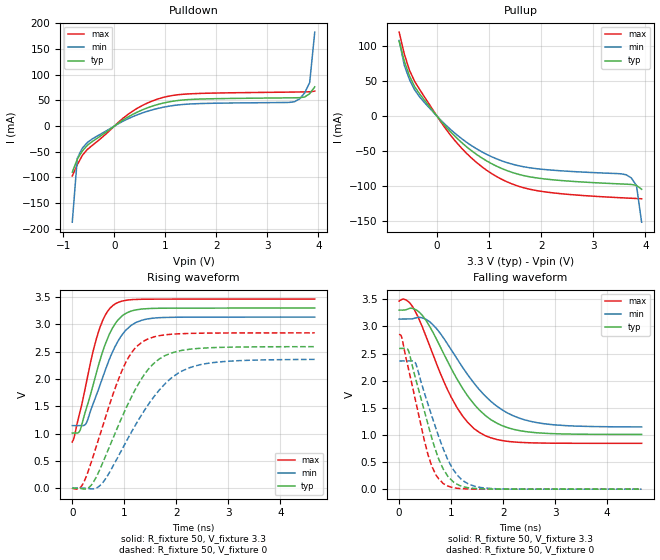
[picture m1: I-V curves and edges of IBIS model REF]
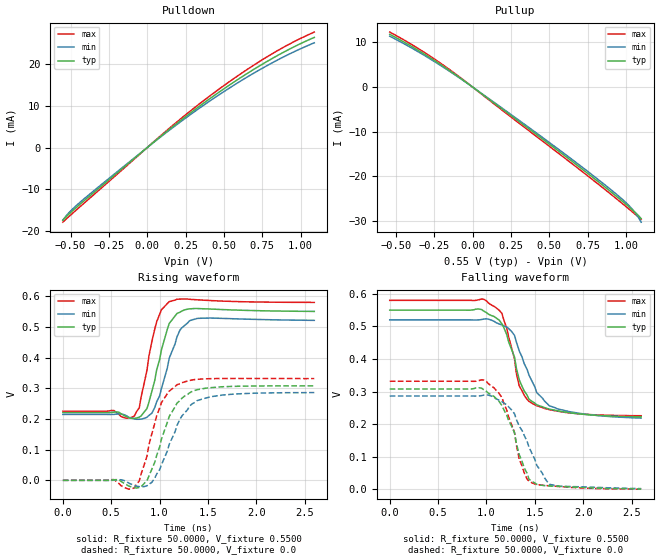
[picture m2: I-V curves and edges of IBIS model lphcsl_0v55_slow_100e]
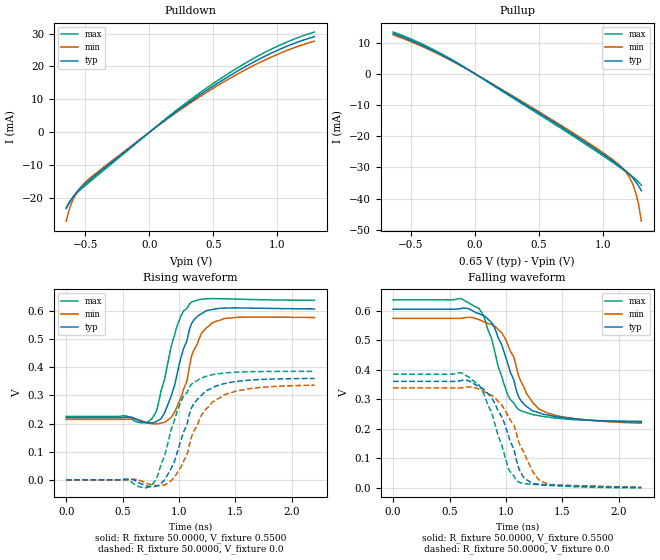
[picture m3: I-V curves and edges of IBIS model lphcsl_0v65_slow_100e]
| Integrated Devices Technolgy, Inc
[IBIS Ver]   4.1
[File name]   9fgl06p1.ibs
[File Rev]   1.0
|Rev history   1.0   original ibis data
[Date]   22 March, 2016
[Disclaimer] Integrated Device Technology, Inc. ("IDT") hereby grants the
   user of this ibis model a non-exclusive, nontransferable
   license to use this ibis model under the following terms. the
   user is granted this license only to use the ibis model and is
   not granted rights to sell, copy (except as needed to run the
   ibis model), rent, lease or sub-license the ibis model in
   whole or in part, or in modified form to anyone. the user may
   modify the ibis model to suit its specific applications, but
   rights to derivative works and such modifications shall belong
   to idt. this ibis model is provided on an as is" basis and idt
   makes absolutely no warranty with respect to the information
   contained herein. idt disclaims and customer waives all
   warranties, express and implied, including warranties of
   merchantability and fitness for a particular purpose. the
   entire risk as to quality and performance is with the user
   accordingly, in no event shall idt be liable for any direct or
   indirect damages, whether in contract or tort, including any
   lost profits or other incidental, consequential, exemplary, or
   punitive damages arising out of the use or application of the
   ibis model. further, idt reserves the right to make changes
   without notice to any product herein to improve reliability,
   function, or design. idt does not convey any license under
   patent rights or any other intellectual property rights,
   including those of third parties. idt is not obligated to
   provide maintenance or support for the licensed ibis model.
[Copyright]   Copyright 2012, Integrated Devices Technolgy, Inc. all rights
   reserved
[Component]   9fgl06p1
[Manufacturer] Integrated Device Technology, Inc.
[Package]
R_pkg   72.4655m   58.886m   86.045m
L_pkg   1.47175nH   1.11650nH   1.77850nH
C_pkg   0.07747pF   0.07444pF   0.08050pF
[Pin] signal_name  model_name
1   vSS_EN_tri   GND
2   X1_25   X1
3   X2   X2
4   VDDXTAL3.3   POWER
5   VDDREF3.3   POWER
6   vSADR/REF3.3   REF
7   NC   NC
8   GNDDIG   GND
9   SCLK_3.3   SCIN
10   SDATA_3.3   SCIN
11   VDDDIG3.3   POWER
12   VDDIO   POWER
13   vOE0#   IN
14   DIF0   LP_HCSL
15   DIF0#   LP_HCSL
16   VDD3.3   POWER
17   VDDIO   POWER
18   DIF1   LP_HCSL
19   DIF1#   LP_HCSL
20   NC   NC
21   vOE1#   IN
22   DIF2   LP_HCSL
23   DIF2#   LP_HCSL
24   vOE2#   IN
25   NC   NC
26   VDDA3.3   POWER
27   VDDIO   POWER
28   DIF3   LP_HCSL
29   DIF3#   LP_HCSL
30   vOE3#   IN
31   VDD3.3   POWER
32   VDDIO   POWER
33   DIF4   LP_HCSL
34   DIF4#   LP_HCSL
35   vOE4#   IN
36   DIF5   LP_HCSL
37   DIF5#   LP_HCSL
38   vOE5#   IN
39   VDDIO   POWER
40   ^CKPWRGD_PD#   PD
41   ePAD   GND
[Diff Pin]  inv_pin  vdiff tdelay_typ tdelay_min  tdelay_max
14   15   NA   0   0   0
18   19   NA   0   0   0
22   23   NA   0   0   0
28   29   NA   0   0   0
33   34   NA   0   0   0
36   37   NA   0   0   0
[Model Selector] LP_HCSL
lphcsl_0v55_fast_33e amplitude 0.55V, slew rate fast, 33 ohm diff impedance
lphcsl_0v55_slow_33e amplitude 0.55V, slew rate slow, 33 ohm diff impedance
lphcsl_0v65_fast_33e amplitude 0.65V, slew rate fast, 33 ohm diff impedance
lphcsl_0v65_slow_33e amplitude 0.65V, slew rate slow, 33 ohm diff impedance
lphcsl_0v70_fast_33e amplitude 0.70V, slew rate fast, 33 ohm diff impedance
lphcsl_0v70_slow_33e amplitude 0.70V, slew rate slow, 33 ohm diff impedance
lphcsl_0v80_fast_33e amplitude 0.80V, slew rate fast, 33 ohm diff impedance
lphcsl_0v80_slow_33e amplitude 0.80V, slew rate slow, 33 ohm diff impedance
lphcsl_0v55_fast_85e amplitude 0.55V, slew rate fast, 85 ohm diff impedance
lphcsl_0v55_slow_85e amplitude 0.55V, slew rate slow, 85 ohm diff impedance
lphcsl_0v65_fast_85e amplitude 0.65V, slew rate fast, 85 ohm diff impedance
lphcsl_0v65_slow_85e amplitude 0.65V, slew rate slow, 85 ohm diff impedance
lphcsl_0v70_fast_85e amplitude 0.70V, slew rate fast, 85 ohm diff impedance
lphcsl_0v70_slow_85e amplitude 0.70V, slew rate slow, 85 ohm diff impedance
lphcsl_0v80_fast_85e amplitude 0.80V, slew rate fast, 85 ohm diff impedance
lphcsl_0v80_slow_85e amplitude 0.80V, slew rate slow, 85 ohm diff impedance
lphcsl_0v55_fast_100e amplitude 0.55V, slew rate fast, 100 ohm diff impedance
lphcsl_0v55_slow_100e amplitude 0.55V, slew rate slow, 100 ohm diff impedance
lphcsl_0v65_fast_100e amplitude 0.65V, slew rate fast, 100 ohm diff impedance
lphcsl_0v65_slow_100e amplitude 0.65V, slew rate slow, 100 ohm diff impedance
lphcsl_0v70_fast_100e amplitude 0.70V, slew rate fast, 100 ohm diff impedance
lphcsl_0v70_slow_100e amplitude 0.70V, slew rate slow, 100 ohm diff impedance
lphcsl_0v80_fast_100e amplitude 0.80V, slew rate fast, 100 ohm diff impedance
lphcsl_0v80_slow_100e amplitude 0.80V, slew rate slow, 100 ohm diff impedance
| Models and submodels in the file (30): REF (Output), lphcsl_0v55_fast_100e (Output), lphcsl_0v55_slow_100e (Output), lphcsl_0v65_fast_100e (Output), lphcsl_0v65_slow_100e (Output), lphcsl_0v70_fast_100e (Output), lphcsl_0v70_slow_100e (Output), lphcsl_0v80_fast_100e (Output), lphcsl_0v80_slow_100e (Output), lphcsl_0v55_fast_85e (Output), lphcsl_0v55_slow_85e (Output), lphcsl_0v65_fast_85e (Output), lphcsl_0v65_slow_85e (Output), lphcsl_0v70_fast_85e (Output), lphcsl_0v70_slow_85e (Output), lphcsl_0v80_fast_85e (Output), lphcsl_0v80_slow_85e (Output), lphcsl_0v55_fast_33e (Output), lphcsl_0v55_slow_33e (Output), lphcsl_0v65_fast_33e (Output), lphcsl_0v65_slow_33e (Output), lphcsl_0v70_fast_33e (Output), lphcsl_0v70_slow_33e (Output), lphcsl_0v80_fast_33e (Output), lphcsl_0v80_slow_33e (Output), SCIN (Input), IN (Input), PD (Input), X1 (Input), X2 (Output)
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[Model]   REF
Model_type   Output
Polarity   Non-Inverting
|   typ   min   max
C_comp   2pF   1.5pF   2.5pF
Vmeas = 1.65V
Rref = 50
Cref = 0
Vref = 1.65V
|   typ   min   max
[Voltage range]   3.3V   3.135V   3.465V
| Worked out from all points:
|   slope of the pulldown table from 0 to 0.495 V, typ, clamps not added: 16.9 ohm
|   slope of the pullup table from 0 to 0.495 V, typ, clamps not added: 12.6 ohm
|   rising waveform, R_fixture 50, V_fixture 3.3: 20-80 % time 450ps typ, 507ps min, 388ps max; typ from 1.01 V to 3.3 V
|   falling waveform, R_fixture 50, V_fixture 3.3: 20-80 % time 857ps typ, 970ps min, 739ps max; typ from 3.3 V to 1.01 V
|   rising waveform, R_fixture 50, V_fixture 0: 20-80 % time 771ps typ, 936ps min, 618ps max; typ from 0 V to 2.59 V
|   falling waveform, R_fixture 50, V_fixture 0: 20-80 % time 472ps typ, 527ps min, 413ps max; typ from 2.59 V to 0 V
[Pulldown]
|Voltage   I (typ)   I (min)   I (max)
|Note, modeling breaks down at 250mA and above.  This is well beyond the functional   |
|operating range of the device.  Should this scenario occur, catastrophic failure and   |
|possible damage to the device and/or board is of higher concern than the I-V curve   |
|behavior.  The IBIS checker will flag currents in excess of 10A with warnings.  Lines   |
|with currents in excess of 0.35 A have been commented out.  The points still remain|
|available to the user if the user desires to use them.   |
|-3.30000e+00   -4.58626e+02   -3.98855e+02   -5.58913e+02
|-3.20100e+00   -4.38670e+02   -3.81813e+02   -5.34126e+02
|-3.10200e+00   -4.18718e+02   -3.64776e+02   -5.09343e+02
|-3.00300e+00   -3.98770e+02   -3.47745e+02   -4.84563e+02
|-2.90400e+00   -3.78827e+02   -3.30720e+02   -4.59787e+02
|-2.80500e+00   -3.58890e+02   -3.13701e+02   -4.35015e+02
|-2.70600e+00   -3.38959e+02   -2.96690e+02   -4.10248e+02
|-2.60700e+00   -3.19035e+02   -2.79688e+02   -3.85486e+02
|-2.50800e+00   -2.99119e+02   -2.62696e+02   -3.60731e+02
|-2.40900e+00   -2.79213e+02   -2.45715e+02   -3.35984e+02
|-2.31000e+00   -2.59319e+02   -2.28747e+02   -3.11245e+02
|-2.21100e+00   -2.39437e+02   -2.11796e+02   -2.86516e+02
|-2.11200e+00   -2.19572e+02   -1.94864e+02   -2.61800e+02
|-2.01300e+00   -1.99726e+02   -1.77955e+02   -2.37100e+02
|-1.91400e+00   -1.79905e+02   -1.61075e+02   -2.12419e+02
|-1.81500e+00   -1.60116e+02   -1.44233e+02   -1.87763e+02
|-1.71600e+00   -1.40369e+02   -1.27441e+02   -1.63140e+02
|-1.61700e+00   -1.20682e+02   -1.10717e+02   -1.38565e+02
|-1.51800e+00   -1.01080e+02   -9.40899e+01   -1.14061e+02
|-1.41900e+00   -8.16135e+01   -7.76121e+01   -8.96701e+01
|-1.32000e+00   -6.23864e+01   -6.13830e+01   -6.54941e+01
|-1.22100e+00   -4.36066e+01   -4.55730e+01   -4.17841e+01
|-1.12200e+00   -2.55446e+01   -3.03740e+01   -1.89497e+01
|-1.02300e+00   -8.13369e+00   -1.57511e+01   -1.01906e+00
|-9.24000e-01   -3.55892e-01   -2.38948e+00   -1.27879e-01
-825mV    -89.74mA   -186.9mA   -97.05mA
-726mV    -64.34mA   -62.46mA   -75.03mA
-627mV    -48.3mA    -42.65mA   -56.86mA
-528mV    -37.22mA   -31.89mA   -45.33mA
363mV     22.88mA    18.45mA    29.33mA
957mV     44.74mA    36.62mA    55.73mA
1.551V    52.05mA    43.3mA     63.04mA
3.531V    55.03mA    47.39mA    66.19mA
3.63V     55.21mA    52.95mA    66.32mA
3.729V    56.59mA    64.36mA    66.46mA
3.828V    63.02mA    84.81mA    66.64mA
3.927V    76.26mA    182.8mA    67.99mA
| 4.02600e+00   9.63336e-02   1.95544e+00   7.56685e-02
| 4.12500e+00   1.29319e-01   1.96109e+01   9.19025e-02
| 4.22400e+00   6.62462e-01   4.21550e+01   1.15435e-01
| 4.32300e+00   1.51637e+01   6.47670e+01   1.37492e-01
| 4.42200e+00   4.22442e+01   8.74545e+01   2.35006e-01
| 4.52100e+00   6.94172e+01   1.10195e+02   8.92943e+00
| 4.62000e+00   9.66780e+01   1.32968e+02   4.35589e+01
| 4.71900e+00   1.23991e+02   1.55761e+02   7.83218e+01
| 4.81800e+00   1.51333e+02   1.78569e+02   1.13180e+02
| 4.91700e+00   1.78693e+02   2.01386e+02   1.48085e+02
| 5.01600e+00   2.06065e+02   2.24210e+02   1.83014e+02
| 5.11500e+00   2.33446e+02   2.47041e+02   2.17958e+02
| 5.21400e+00   2.60834e+02   2.69877e+02   2.52912e+02
| 5.31300e+00   2.88228e+02   2.92717e+02   2.87874e+02
| 5.41200e+00   3.15625e+02   3.15560e+02   3.22841e+02
| 5.51100e+00   3.43027e+02   3.38407e+02   3.57813e+02
| 5.61000e+00   3.70432e+02   3.61256e+02   3.92789e+02
| 5.70900e+00   3.97841e+02   3.84108e+02   4.27769e+02
| 5.80800e+00   4.25252e+02   4.06963e+02   4.62752e+02
| 5.90700e+00   4.52666e+02   4.29821e+02   4.97738e+02
| 6.00600e+00   4.80082e+02   4.52680e+02   5.32727e+02
| 6.10500e+00   5.07501e+02   4.75543e+02   5.67718e+02
| 6.20400e+00   5.34922e+02   4.98407e+02   6.02711e+02
| 6.30300e+00   5.62345e+02   5.21273e+02   6.37705e+02
| 6.40200e+00   5.89770e+02   5.44142e+02   6.72701e+02
| 6.50100e+00   6.17197e+02   5.67013e+02   7.07699e+02
| 6.60000e+00   6.44626e+02   5.89886e+02   7.42698e+02
[Pullup]
|Voltage   I (typ)   I (min)   I (max)
|Note, modeling breaks down at 250mA and above.  This is well beyond the functional   |
|operating range of the device.  Should this scenario occur, catastrophic failure and   |
|possible damage to the device and/or board is of higher concern than the I-V curve   |
|behavior.  The IBIS checker will flag currents in excess of 10A with warnings.  Lines   |
|with currents in excess of 0.35 A have been commented out.  The points still remain|
|available to the user if the user desires to use them.   |
|-3.30000e+00   6.44680e+02   5.51825e+02   8.01095e+02
|-3.20100e+00   6.17254e+02   5.28958e+02   7.66095e+02
|-3.10200e+00   5.89830e+02   5.06093e+02   7.31096e+02
|-3.00300e+00   5.62407e+02   4.83230e+02   6.96098e+02
|-2.90400e+00   5.34987e+02   4.60368e+02   6.61102e+02
|-2.80500e+00   5.07568e+02   4.37509e+02   6.26108e+02
|-2.70600e+00   4.80150e+02   4.14651e+02   5.91115e+02
|-2.60700e+00   4.52735e+02   3.91796e+02   5.56124e+02
|-2.50800e+00   4.25322e+02   3.68942e+02   5.21136e+02
|-2.40900e+00   3.97911e+02   3.46091e+02   4.86149e+02
|-2.31000e+00   3.70503e+02   3.23243e+02   4.51165e+02
|-2.21100e+00   3.43097e+02   3.00397e+02   4.16183e+02
|-2.11200e+00   3.15694e+02   2.77554e+02   3.81204e+02
|-2.01300e+00   2.88295e+02   2.54715e+02   3.46229e+02
|-1.91400e+00   2.60900e+02   2.31881e+02   3.11257e+02
|-1.81500e+00   2.33510e+02   2.09052e+02   2.76290e+02
|-1.71600e+00   2.06127e+02   1.86229e+02   2.41329e+02
|-1.61700e+00   1.78751e+02   1.63415e+02   2.06375e+02
|-1.51800e+00   1.51388e+02   1.40613e+02   1.71432e+02
|-1.41900e+00   1.24042e+02   1.17829e+02   1.36506e+02
|-1.32000e+00   9.67252e+01   9.50724e+01   1.01609e+02
|-1.22100e+00   6.94599e+01   7.23604e+01   6.67700e+01
|-1.12200e+00   4.22820e+01   4.97173e+01   3.20469e+01
|-1.02300e+00   1.51962e+01   2.71494e+01   2.11287e+00
|-9.24000e-01   6.89030e-01   5.34223e+00   1.97623e-01
|-8.25000e-01   1.48916e-01   3.54714e-01   1.54087e-01
-726mV    106.9mA    108.2mA    120.1mA
-627mV    78.63mA    72.64mA    88.74mA
-528mV    57.36mA    52.3mA     65.5mA
-330mV    31.45mA    27.24mA    37.82mA
363mV     -30.02mA   -25.58mA   -36.52mA
957mV     -64.05mA   -54.65mA   -77.43mA
1.353V    -77.99mA   -66.51mA   -94.06mA
1.848V    -87.45mA   -74.38mA   -105.4mA
3.63V     -97.08mA   -83.63mA   -116.9mA
3.729V    -97.47mA   -88.18mA   -117.2mA
3.828V    -98.9mA    -99mA      -117.5mA
3.927V    -104.4mA   -151.4mA   -117.9mA
| 4.02600e+00   -1.15410e-01   -9.65481e-01   -1.19366e-01
| 4.12500e+00   -1.36603e-01   -1.09884e+01   -1.26324e-01
| 4.22400e+00   -3.99361e-01   -2.54841e+01   -1.40663e-01
| 4.32300e+00   -8.17474e+00   -4.04654e+01   -1.58277e-01
| 4.42200e+00   -2.55843e+01   -5.60873e+01   -2.17491e-01
| 4.52100e+00   -4.36450e+01   -7.21990e+01   -4.28595e+00
| 4.62000e+00   -6.24226e+01   -8.86071e+01   -2.64922e+01
| 4.71900e+00   -8.16508e+01   -1.05189e+02   -4.96573e+01
| 4.81800e+00   -1.01115e+02   -1.21884e+02   -7.35635e+01
| 4.91700e+00   -1.20715e+02   -1.38656e+02   -9.78285e+01
| 5.01600e+00   -1.40403e+02   -1.55482e+02   -1.22263e+02
| 5.11500e+00   -1.60149e+02   -1.72350e+02   -1.46794e+02
| 5.21400e+00   -1.79938e+02   -1.89250e+02   -1.71387e+02
| 5.31300e+00   -1.99760e+02   -2.06175e+02   -1.96022e+02
| 5.41200e+00   -2.19606e+02   -2.23121e+02   -2.20688e+02
| 5.51100e+00   -2.39472e+02   -2.40084e+02   -2.45378e+02
| 5.61000e+00   -2.59355e+02   -2.57061e+02   -2.70086e+02
| 5.70900e+00   -2.79251e+02   -2.74051e+02   -2.94808e+02
| 5.80800e+00   -2.99159e+02   -2.91052e+02   -3.19543e+02
| 5.90700e+00   -3.19077e+02   -3.08062e+02   -3.44288e+02
| 6.00600e+00   -3.39003e+02   -3.25080e+02   -3.69042e+02
| 6.10500e+00   -3.58937e+02   -3.42106e+02   -3.93803e+02
| 6.20400e+00   -3.78878e+02   -3.59138e+02   -4.18571e+02
| 6.30300e+00   -3.98826e+02   -3.76177e+02   -4.43346e+02
| 6.40200e+00   -4.18779e+02   -3.93221e+02   -4.68125e+02
| 6.50100e+00   -4.38737e+02   -4.10271e+02   -4.92910e+02
| 6.60000e+00   -4.58699e+02   -4.27325e+02   -5.17700e+02
[Ramp]
|   typ   min   max
dV/dt_r   1.566/0.774n   1.425/0.94n   1.718/0.621n
dV/dt_f   1.396/0.866n   1.212/0.979n   1.595/0.746n
R_load =   50
[Rising Waveform]
R_fixture = 50
V_fixture = 3.3   |Vcc_typ
V_fixture_min = 3.135 |Vcc_min
V_fixture_max = 3.465 |Vcc_max
C_fixture = 0.0p
| Time   typ   min   max
0s        1.008V     1.145V     844.6mV
34.71ps   1.008V     1.145V     923.1mV
154.3ps   1.071V     1.145V     1.413V
275.2ps   1.472V     1.202V     1.956V
479.5ps   2.168V     1.745V     2.789V
635.5ps   2.641V     2.166V     3.174V
823.7ps   3.01V      2.596V     3.375V
1.129ns   3.244V     2.981V     3.453V
1.433ns   3.289V     3.099V     3.463V
4.662ns   3.3V       3.135V     3.465V
[Falling Waveform]
R_fixture = 50
V_fixture = 3.3   |Vcc_typ
V_fixture_min = 3.135 |Vcc_min
V_fixture_max = 3.465 |Vcc_max
C_fixture = 0.0p
| Time   typ   min   max
0s        3.3V       3.135V     3.465V
120.3ps   3.304V     3.135V     3.493V
247.8ps   3.333V     3.138V     3.377V
425ps     3.225V     3.162V     3.038V
624.4ps   2.937V     3.054V     2.545V
1.111ns   2.034V     2.407V     1.506V
1.539ns   1.462V     1.838V     1.048V
1.979ns   1.171V     1.463V     896.3mV
2.515ns   1.052V     1.252V     854.4mV
4.666ns   1.008V     1.146V     844.6mV
[Rising Waveform]
R_fixture = 50
V_fixture = 0
C_fixture = 0.0p
| Time   typ   min   max
0s        23.89nV    60.43nV    30.4nV
191.1ps   -13.44mV   129.7uV    54.48mV
415.8ps   124mV      -13.01mV   625.4mV
623.1ps   548.9mV    147.1mV    1.254V
939.4ps   1.267V     680mV      2.117V
1.156ns   1.708V     1.059V     2.505V
1.348ns   2.027V     1.367V     2.681V
1.787ns   2.43V      1.916V     2.809V
2.339ns   2.554V     2.232V     2.838V
4.662ns   2.593V     2.359V     2.845V
[Falling Waveform]
R_fixture = 50
V_fixture = 0
C_fixture = 0.0p
| Time   typ   min   max
0s        2.593V     2.362V     2.845V
47.92ps   2.593V     2.362V     2.804V
169.8ps   2.571V     2.362V     2.258V
309ps     2.063V     2.332V     1.656V
482.9ps   1.445V     1.783V     905.2mV
624.2ps   958.6mV    1.36V      434.3mV
847.8ps   371.4mV    743.3mV    103.8mV
1.113ns   93.12mV    264.4mV    16.96mV
1.53ns    8.102mV    37.41mV    1.012mV
4.662ns   -1.039uV   -794nV     -867.7nV
[Model]   lphcsl_0v55_slow_100e
Model_type Output
Polarity   Non-Inverting
Enable   Active-High
Vmeas =  0.4000V
Cref =   2.0000pF
Rref =   0.0
Vref =   0.4000V
C_comp   1.1000pF   1.0000pF   1.2000pF
[Temperature Range]   25.0000   85.0000   -40.0000
[Voltage Range]   0.5500V   0.5200V   0.5800V
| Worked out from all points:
|   slope of the pulldown table from 0 to 0.083 V, typ, clamps not added: 32.7 ohm
|   slope of the pullup table from 0 to 0.083 V, typ, clamps not added: 39.3 ohm
|   rising waveform, R_fixture 50.0000, V_fixture 0.5500: 20-80 % time 156ps typ, 172ps min, 137ps max; typ from 0.221 V to 0.551 V
|   rising waveform, R_fixture 50.0000, V_fixture 0.0: 20-80 % time 218ps typ, 257ps min, 187ps max; typ from 0 V to 0.308 V
|   falling waveform, R_fixture 50.0000, V_fixture 0.5500: 20-80 % time 226ps typ, 279ps min, 186ps max; typ from 0.55 V to 0.222 V
|   falling waveform, R_fixture 50.0000, V_fixture 0.0: 20-80 % time 221ps typ, 262ps min, 196ps max; typ from 0.308 V to 0.001 V
[Pulldown]
|Voltage   I(typ)   I(min)   I(max)
-550mV    -17.42mA   -17.37mA   -17.87mA
-510mV    -15.92mA   -15.58mA   -16.5mA
-470mV    -14.59mA   -14.14mA   -15.2mA
-350mV    -10.82mA   -10.4mA    -11.34mA
70mV      2.144mA    2.042mA    2.274mA
330mV     9.616mA    9.161mA    10.17mA
550mV     15.31mA    14.58mA    16.15mA
730mV     19.51mA    18.57mA    20.56mA
910mV     23.24mA    22.1mA     24.45mA
1.09V     26.39mA    25.1mA     27.67mA
[Pullup]
|Voltage   I(typ)   I(min)   I(max)
-540mV    11.78mA    11.36mA    12.28mA
-360mV    8.313mA    7.995mA    8.73mA
-160mV    3.912mA    3.748mA    4.141mA
40mV      -1.02mA    -975.2uA   -1.083mA
480mV     -12.23mA   -11.87mA   -12.71mA
760mV     -19.55mA   -19.1mA    -20.1mA
960mV     -25.05mA   -24.6mA    -25.58mA
1.04V     -27.39mA   -27.24mA   -27.85mA
1.08V     -28.69mA   -29.05mA   -29.01mA
1.1V      -29.42mA   -30.23mA   -29.61mA
[Ramp]
| variable   typ   min   max
dV/dt_r  0.1848/0.2190n   0.1717/0.2485n   0.1991/0.1882n
dV/dt_f  0.1965/0.2484n   0.1808/0.2865n   0.2125/0.2078n
R_load = 50.0000
[Rising Waveform]
R_fixture= 50.0000
V_fixture= 0.5500
V_fixture_min= 0.5200
V_fixture_max= 0.5800
|time   V(typ)   V(min)   V(max)
0s        221mV      214.9mV    225.3mV
740ps     201.9mV    200.2mV    210mV
790ps     206mV      199.1mV    236.4mV
870ps     234.3mV    205.7mV    359.2mV
920ps     290mV      218.6mV    452mV
1.02ns    426.3mV    299.8mV    556.5mV
1.1ns     511.8mV    398.5mV    582.6mV
1.21ns    548.2mV    489.5mV    591.1mV
1.39ns    560.3mV    528.2mV    588.8mV
2.6ns     550.9mV    521.7mV    580.3mV
[Rising Waveform]
R_fixture= 50.0000
V_fixture= 0.0
V_fixture_min= 0.0
V_fixture_max= 0.0
|time   V(typ)   V(min)   V(max)
0s        0V         0V         0V
550ps     2.324mV    951.5uV    -2.512mV
740ps     -24.18mV   -16.37mV   -24.55mV
790ps     -23.47mV   -20.51mV   -2.409mV
920ps     36.17mV    -6.753mV   151.8mV
1.02ns    135mV      51.17mV    253.8mV
1.18ns    251.8mV    179.1mV    311.9mV
1.31ns    285.3mV    242.2mV    325.5mV
1.52ns    302mV      272.4mV    331.5mV
2.6ns     308mV      286.1mV    331.8mV
[Falling Waveform]
R_fixture= 50.0000
V_fixture= 0.5500
V_fixture_min= 0.5200
V_fixture_max= 0.5800
|time   V(typ)   V(min)   V(max)
0s        550mV      520mV      580mV
970ps     547.5mV    522.6mV    583.6mV
1.16ns    508mV      504.6mV    540.1mV
1.29ns    406.3mV    472.7mV    400.4mV
1.31ns    370.9mV    451.9mV    355.2mV
1.34ns    335.5mV    423.9mV    316.5mV
1.44ns    276.5mV    350.4mV    269.9mV
1.52ns    259.5mV    296.8mV    256.6mV
1.65ns    246.1mV    256.4mV    244.6mV
2.6ns     222.5mV    218.6mV    225.8mV
[Falling Waveform]
R_fixture= 50.0000
V_fixture= 0.0
V_fixture_min= 0.0
V_fixture_max= 0.0
|time   V(typ)   V(min)   V(max)
0s        307.9mV    286.4mV    331.7mV
970ps     306.1mV    289.1mV    335.8mV
1.16ns    257.3mV    269.1mV    282mV
1.29ns    173.9mV    232mV      174.5mV
1.34ns    105.8mV    193.4mV    91.43mV
1.39ns    66.68mV    165.9mV    50.82mV
1.44ns    31.41mV    129mV      24.81mV
1.52ns    15.24mV    73.8mV     14.68mV
1.65ns    10.13mV    15.34mV    10.72mV
2.6ns     993.4uV    2.118mV    402uV
[Model]   lphcsl_0v65_slow_100e
Model_type Output
Polarity   Non-Inverting
Enable   Active-High
Vmeas =  0.4000V
Cref =   2.0000pF
Rref =   0.0
Vref =   0.4000V
C_comp   1.1000pF   1.0000pF   1.2000pF
[Temperature Range]   25.0000   85.0000   -40.0000
[Voltage Range]   0.6500V   0.6200V   0.6800V
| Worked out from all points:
|   slope of the pulldown table from 0 to 0.098 V, typ, clamps not added: 32.8 ohm
|   slope of the pullup table from 0 to 0.098 V, typ, clamps not added: 40 ohm
|   rising waveform, R_fixture 50.0000, V_fixture 0.5500: 20-80 % time 158ps typ, 170ps min, 154ps max; typ from 0.221 V to 0.607 V
|   rising waveform, R_fixture 50.0000, V_fixture 0.0: 20-80 % time 204ps typ, 240ps min, 203ps max; typ from 0 V to 0.36 V
|   falling waveform, R_fixture 50.0000, V_fixture 0.5500: 20-80 % time 214ps typ, 239ps min, 199ps max; typ from 0.606 V to 0.223 V
|   falling waveform, R_fixture 50.0000, V_fixture 0.0: 20-80 % time 211ps typ, 241ps min, 199ps max; typ from 0.361 V to 0.001 V
[Pulldown]
|Voltage   I(typ)   I(min)   I(max)
-650mV    -23.23mA   -27.08mA   -22.85mA
-630mV    -21.73mA   -23.92mA   -21.53mA
-610mV    -20.42mA   -21.63mA   -20.41mA
-590mV    -19.28mA   -19.88mA   -19.45mA
-550mV    -17.42mA   -17.37mA   -17.87mA
-510mV    -15.92mA   -15.58mA   -16.5mA
-350mV    -10.82mA   -10.4mA    -11.34mA
130mV     3.938mA    3.75mA     4.173mA
450mV     12.8mA     12.19mA    13.51mA
770mV     20.38mA    19.39mA    21.48mA
1.03V     25.42mA    24.16mA    26.67mA
1.29V     29.08mA    27.71mA    30.47mA
[Pullup]
|Voltage   I(typ)   I(min)   I(max)
-640mV    12.9mA     12.48mA    13.37mA
-340mV    7.668mA    7.369mA    8.057mA
-40mV     988uA      943.5uA    1.052mA
700mV     -17.66mA   -17.23mA   -18.19mA
1.08V     -28.05mA   -27.62mA   -28.49mA
1.16V     -30.49mA   -30.54mA   -30.78mA
1.2V      -31.91mA   -32.71mA   -31.96mA
1.22V     -32.74mA   -34.19mA   -32.58mA
1.24V     -33.69mA   -36.08mA   -33.24mA
1.26V     -34.78mA   -38.62mA   -33.96mA
1.28V     -36.03mA   -42.17mA   -34.78mA
1.3V      -37.46mA   -47.25mA   -35.74mA
[Ramp]
| variable   typ   min   max
dV/dt_r  0.2161/0.2242n   0.2018/0.2534n   0.2312/0.1998n
dV/dt_f  0.2311/0.2438n   0.2145/0.2731n   0.2483/0.2072n
R_load = 50.0000
[Rising Waveform]
R_fixture= 50.0000
V_fixture= 0.5500
V_fixture_min= 0.5200
V_fixture_max= 0.5800
|time   V(typ)   V(min)   V(max)
0s        221mV      214.9mV    225.3mV
760ps     202.3mV    199.7mV    217.4mV
800ps     207mV      199.2mV    244.2mV
870ps     236.6mV    203.8mV    355.1mV
960ps     334.6mV    240.3mV    514.3mV
1.07ns    494.6mV    352mV      609.6mV
1.11ns    554.8mV    438.4mV    631.3mV
1.2ns     590.6mV    521.6mV    641.9mV
1.4ns     610.2mV    573mV      643.4mV
2.2ns     607.2mV    576.7mV    637.9mV
[Rising Waveform]
R_fixture= 50.0000
V_fixture= 0.0
V_fixture_min= 0.0
V_fixture_max= 0.0
|time   V(typ)   V(min)   V(max)
0s        0V         0V         0V
530ps     1.461mV    194.3uV    1.992mV
730ps     -23.41mV   -15.09mV   -26.03mV
800ps     -22.54mV   -20.61mV   3.759mV
960ps     66.54mV    9.62mV     212.7mV
1.07ns    195.9mV    88.33mV    309.7mV
1.13ns    270.3mV    172.7mV    346.1mV
1.24ns    316.7mV    252.3mV    368mV
1.4ns     341.7mV    301.9mV    379.7mV
2.2ns     360.2mV    336.4mV    385.4mV
[Falling Waveform]
R_fixture= 50.0000
V_fixture= 0.5500
V_fixture_min= 0.5200
V_fixture_max= 0.5800
|time   V(typ)   V(min)   V(max)
0s        605.5mV    574.4mV    637mV
600ps     607.9mV    574.5mV    641.2mV
760ps     590.4mV    570.4mV    608.8mV
890ps     550.3mV    550.2mV    479.5mV
980ps     464.9mV    515.1mV    355mV
1.07ns    366.1mV    443.3mV    288.1mV
1.13ns    297.2mV    362.1mV    261.8mV
1.24ns    260.4mV    287.7mV    248.2mV
1.38ns    246.3mV    251.9mV    239.7mV
2.2ns     223.2mV    219.5mV    225.9mV
[Falling Waveform]
R_fixture= 50.0000
V_fixture= 0.0
V_fixture_min= 0.0
V_fixture_max= 0.0
|time   V(typ)   V(min)   V(max)
0s        361mV      338.8mV    385.4mV
600ps     363.4mV    338.9mV    390.1mV
760ps     344.7mV    335.3mV    350.3mV
870ps     307.2mV    315mV      258.9mV
960ps     243.4mV    282.2mV    149mV
1.02ns    179.3mV    243.1mV    67.53mV
1.11ns    70.61mV    159.4mV    20.73mV
1.24ns    14.75mV    53.96mV    11.99mV
1.38ns    10.3mV     11.97mV    8.861mV
2.2ns     1.433mV    2.621mV    465.3uV
